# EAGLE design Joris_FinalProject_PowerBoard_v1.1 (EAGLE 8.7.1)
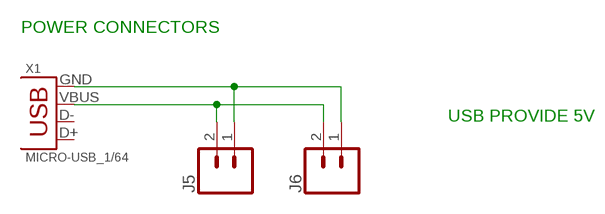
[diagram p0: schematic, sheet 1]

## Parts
J5  CONN_021X02_NO_SILK  [1X02_NO_SILK]
J6  CONN_021X02_NO_SILK  [1X02_NO_SILK]
X1  MICRO-USB_1/64  [DX4R005HJ5_64]

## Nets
N$2: J5.1 J6.1 X1.GND
N$3: J5.2 J6.2 X1.VBUS
Unconnected: X1.D+ X1.D-

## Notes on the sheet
- POWER CONNECTORS
- USB PROVIDE 5V

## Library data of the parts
J5 J6 = SparkFun-Connectors:CONN_02: Multi connection point. Often used as Generic Header-pin footprint for 0.1 inch spaced/style header connections
X1 = fab:MICRO-USB: SMD micro USB connector as found in the fablab inventory. Three footprint variants included: original, as described by manufacturer's datasheet for milling with the 1/100" bit for milling with the 1/64" bit Made by Zaerc.

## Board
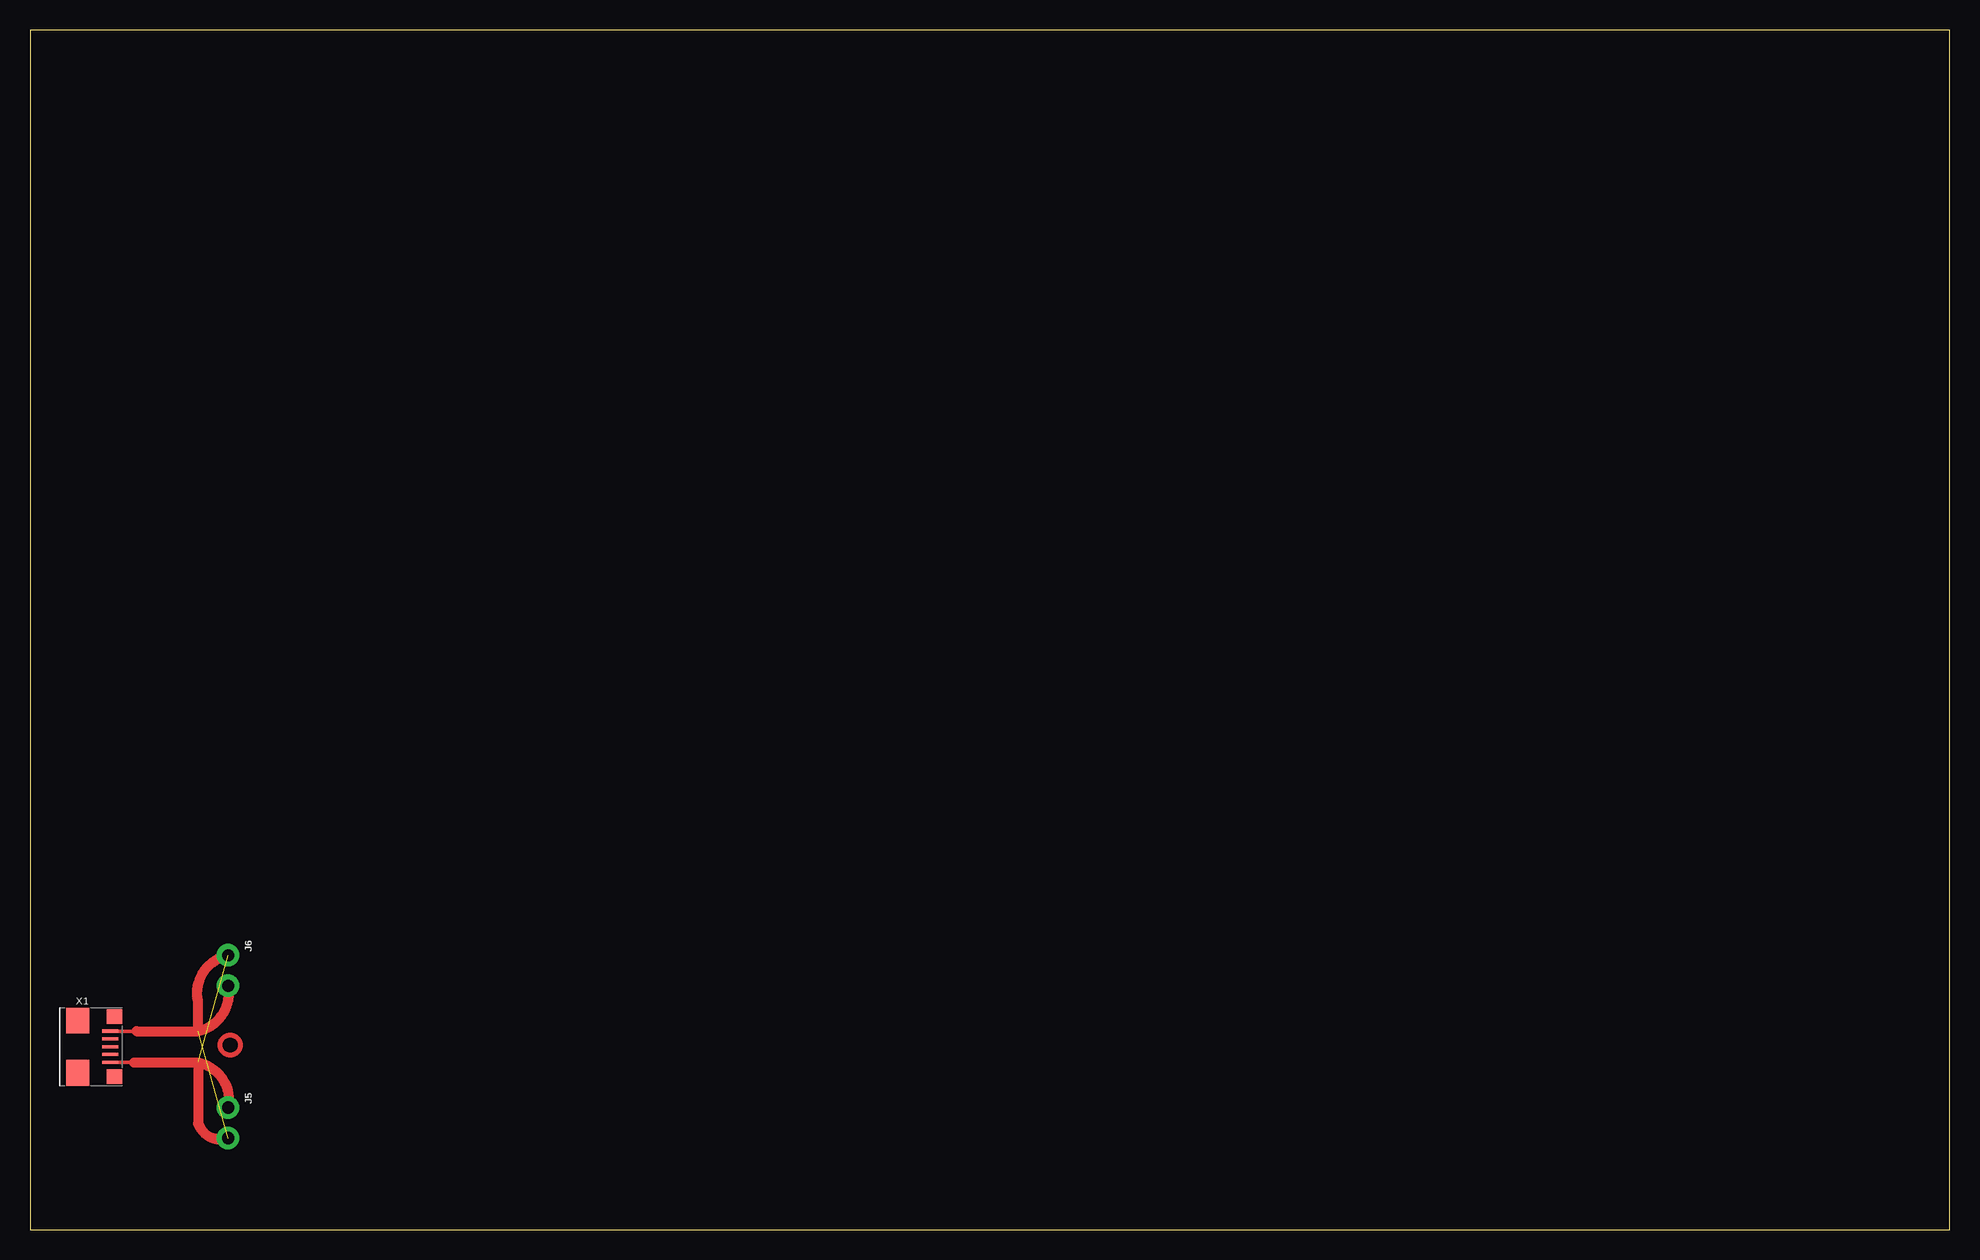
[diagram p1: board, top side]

Size 160 x 100 mm. Coordinates in mm from the lower left corner, seen from the top.
Outline: 0,0 160,0 160,100 0,100 0,0
Copper layers (1*16): Top 0.035mm / dielectric 1.5mm / Bottom 0.035mm
Design rules "default *": minimum track width 6mil, minimum drill 0.35mm, track to track 16mil, track to pad 16mil, pad to pad 16mil, via to via 16mil, smd to smd 16mil, copper to edge 40mil, drill to drill 6mil, minimum pad ring 10mil, minimum via ring 8mil, stop-mask expansion 4mil, vias tented up to drill 0mil, thermal gap 10mil

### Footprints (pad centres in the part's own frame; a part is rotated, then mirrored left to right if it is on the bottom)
1X02_NO_SILK = drill 1.016 pad 1.88: 1 0,0; 2 2.54,0
DX4R005HJ5_64 = smd 0.254 x 1.35: D+ 0,1.6; D- -0.65,1.6; GND 1.3,1.6; ID 0.65,1.6; VBUS -1.3,1.6 | smd 1.2 x 1.3: GND@1 -2.5,1.95; GND@2 2.5,1.95 | smd 2.15 x 1.9: GND@3 -2.175,-1.1; GND@4 2.175,-1.1

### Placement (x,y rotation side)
J5  16.51,10.16 270 top
J6  16.51,22.86 270 top
X1  5.08,15.24 270 top

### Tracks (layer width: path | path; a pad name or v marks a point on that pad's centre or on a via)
N$2  (1 unrouted)
  Top 0.305: X1.GND 8.69,13.92
  Top 0.813: 8.69,13.92 14.02,13.92 | 14.02,13.92 arc-90 J5.1 | 14.02,13.92 14.02,8.84 arc90 16.51,7.62
N$3  (1 unrouted)
  Top 0.305: X1.VBUS 8.86,16.54 arc-90 8.89,16.51
  Top 0.813: 8.86,16.54 14,16.54 | 14,16.54 arc90 J6.2 | 14,16.54 14,19.08 arc-90 16.51,22.86
(copper drawn outside any net)
  shapes: Top circle x1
